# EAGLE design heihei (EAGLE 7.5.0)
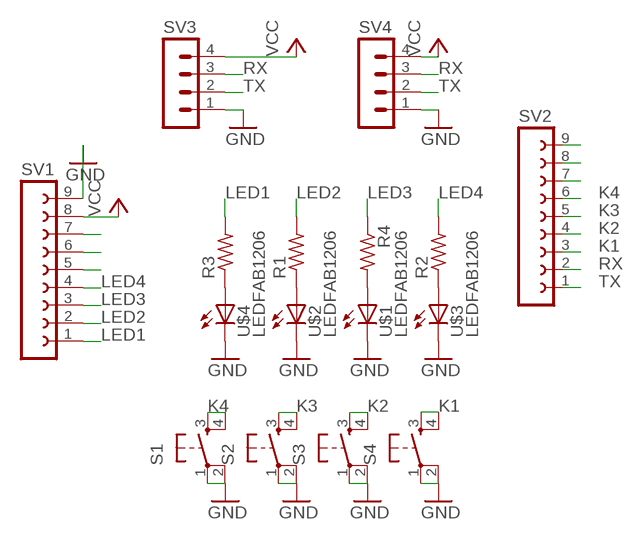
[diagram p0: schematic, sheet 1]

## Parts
R1  RES-US1206FAB  [R1206FAB]
R2  RES-US1206FAB  [R1206FAB]
R3  RES-US1206FAB  [R1206FAB]
R4  RES-US1206FAB  [R1206FAB]
S1  6MM_SWITCH6MM_SWITCH  [6MM_SWITCH]
S2  6MM_SWITCH6MM_SWITCH  [6MM_SWITCH]
S3  6MM_SWITCH6MM_SWITCH  [6MM_SWITCH]
S4  6MM_SWITCH6MM_SWITCH  [6MM_SWITCH]
SV1  FE09-1  [FE09]
SV2  FE09-1  [FE09]
SV3  MA04-1  [MA04-1]
SV4  MA04-1  [MA04-1]
U$1  LEDFAB1206  [LED1206FAB]
U$2  LEDFAB1206  [LED1206FAB]
U$3  LEDFAB1206  [LED1206FAB]
U$4  LEDFAB1206  [LED1206FAB]

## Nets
GND: S1.1(P) S1.2(P1) S2.1(P) S2.2(P1) S3.1(P) S3.2(P1) S4.1(P) S4.2(P1) SV1.9 SV3.1 SV4.1 U$1.2(C) U$2.2(C) U$3.2(C) U$4.2(C)
K1: S4.3(S) S4.4(S1) SV2.3
K2: S3.3(S) S3.4(S1) SV2.4
K3: S2.3(S) S2.4(S1) SV2.5
K4: S1.3(S) S1.4(S1) SV2.6
LED1: R3.2 SV1.1
LED2: R1.2 SV1.2
LED3: R4.1 SV1.3
LED4: R2.2 SV1.4
N$1: SV2.8
N$2: SV2.9
N$3: SV2.7
N$12: SV1.7
N$13: SV1.6
N$18: R3.1 U$4.1(A)
N$19: R1.1 U$2.1(A)
N$20: R4.2 U$1.1(A)
N$21: R2.1 U$3.1(A)
N$22: SV1.5
RX: SV2.2 SV3.3 SV4.3
TX: SV2.1 SV3.2 SV4.2
VCC: SV1.8 SV3.4 SV4.4

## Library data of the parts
R1-R4 = fab:RES-US: Resistor (US Symbol)
S1-S4 = fab:6MM_SWITCH: OMRON SWITCH
SV1 SV2 = con-lsta:FE09-1: FEMALE HEADER; OC_FARNELL: unknown; OC_NEWARK: unknown
SV3 SV4 = con-lstb:MA04-1: PIN HEADER; OC_FARNELL: unknown; OC_NEWARK: unknown
U$1-U$4 = fab:LED: LED

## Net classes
0 default: clearance 0.205 mm

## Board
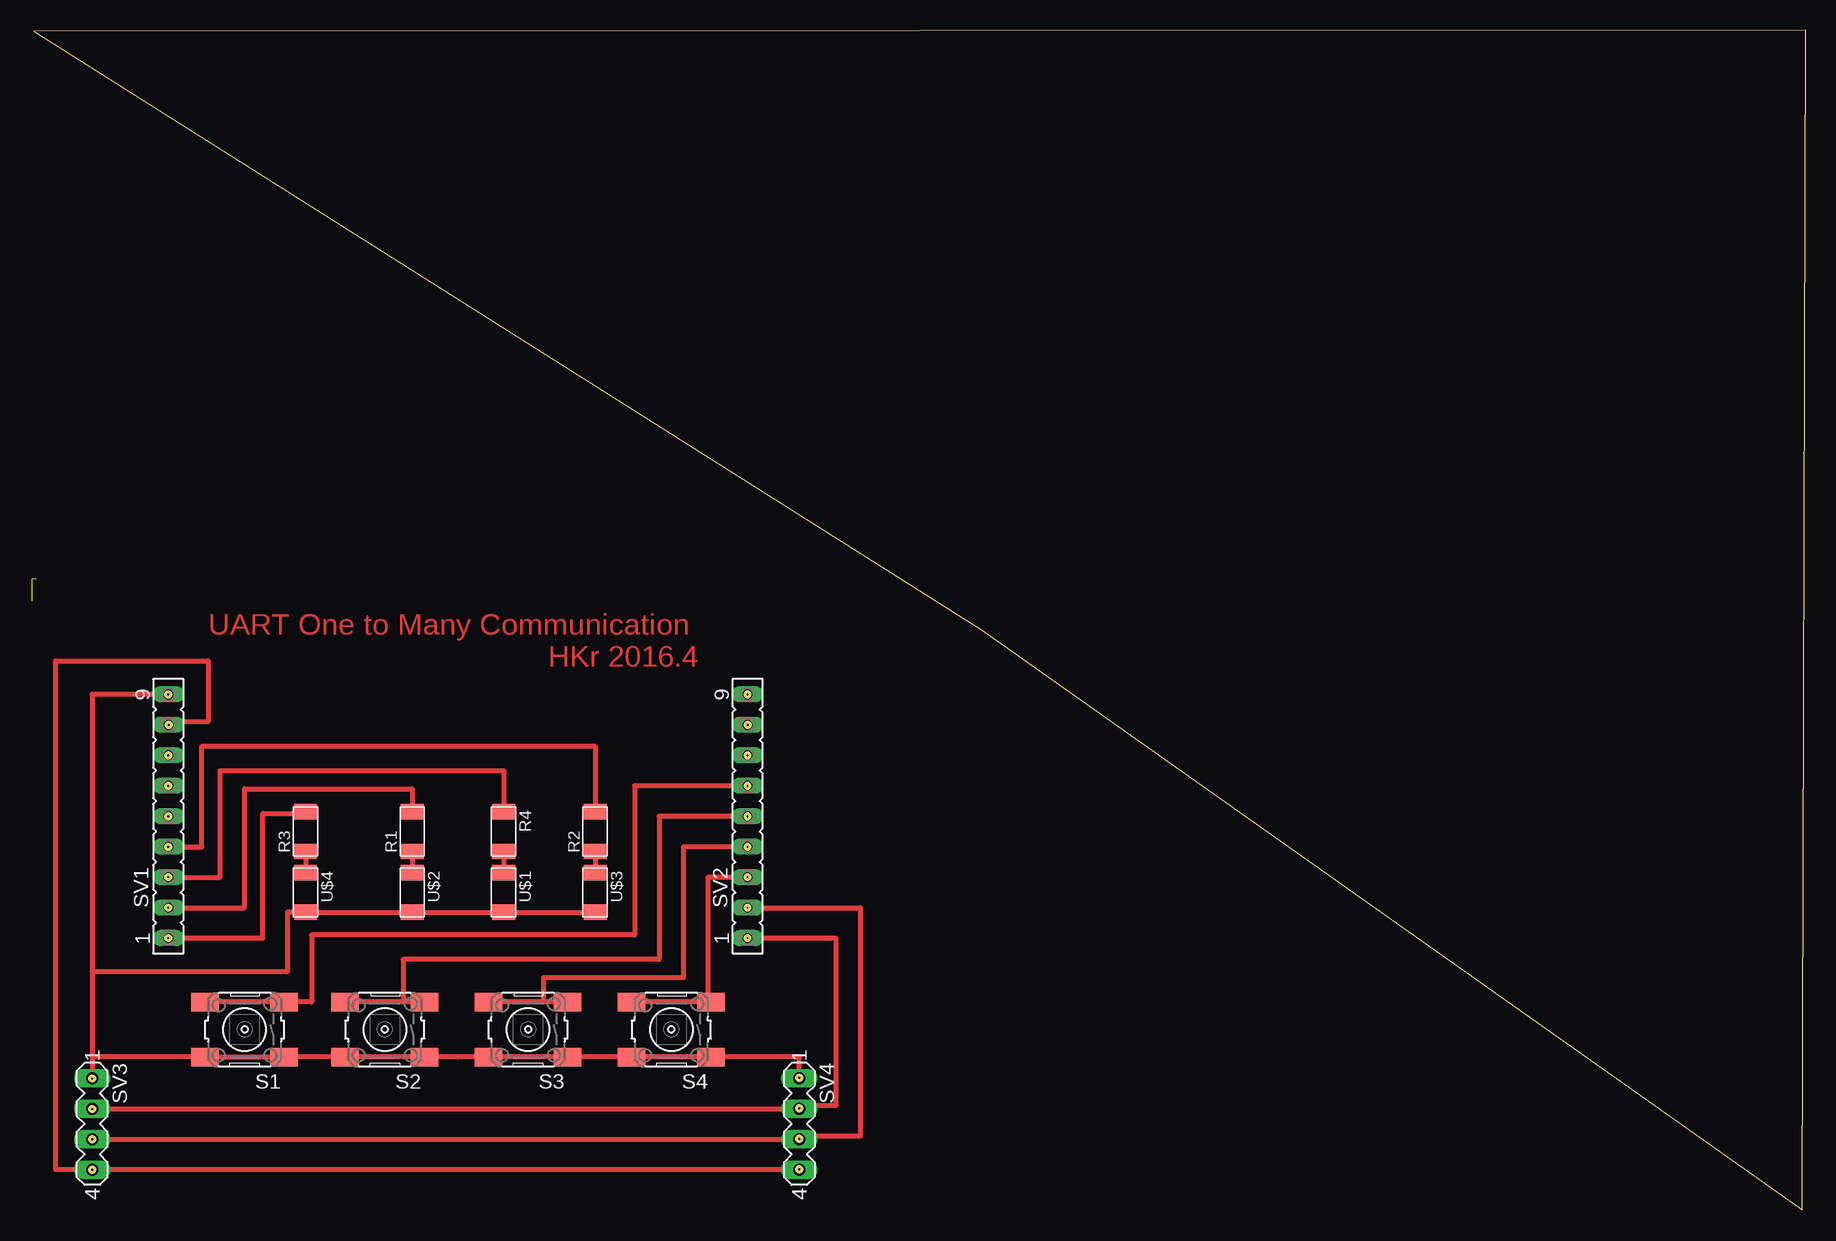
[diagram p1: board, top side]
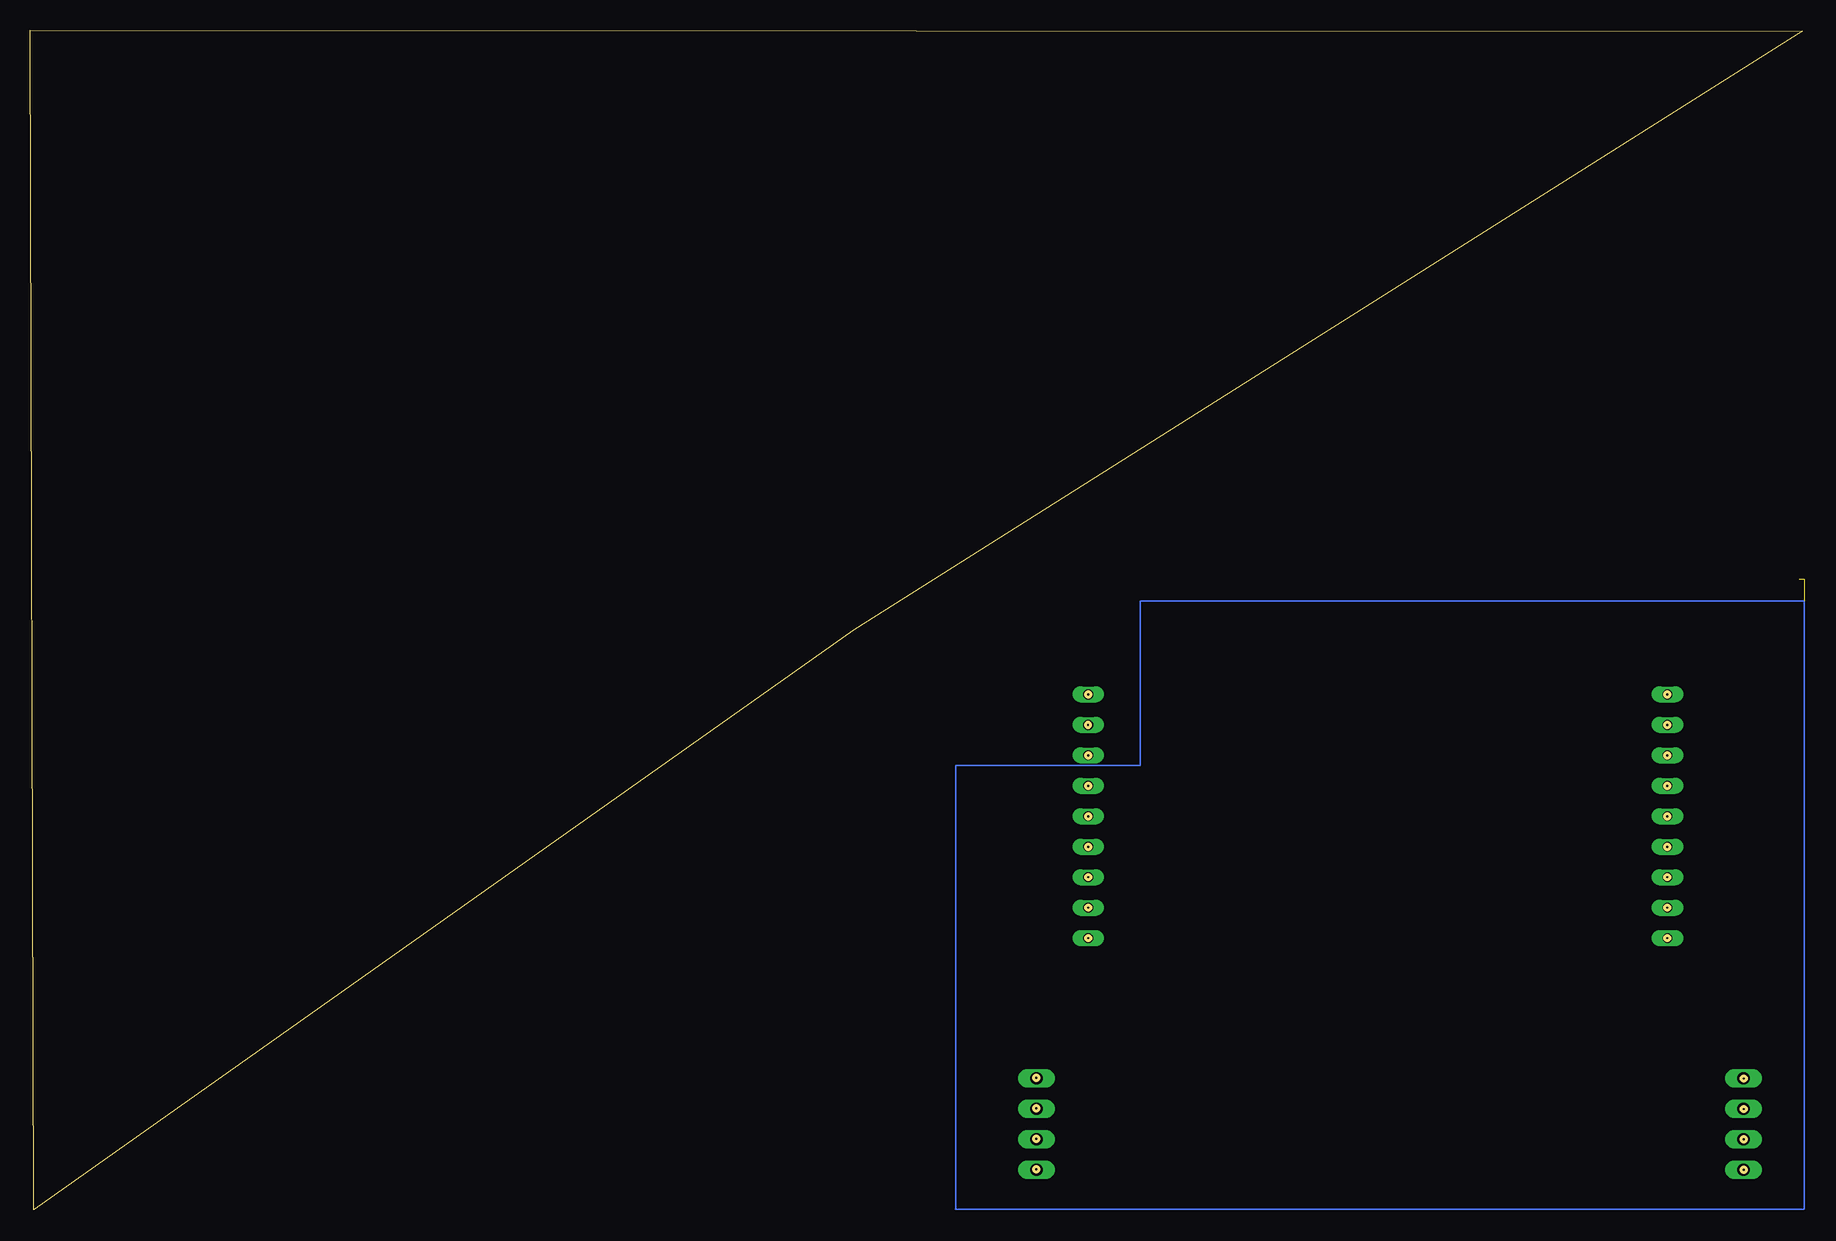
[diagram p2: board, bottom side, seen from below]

Size 147.68 x 98.36 mm. Coordinates in mm from the lower left corner, seen from the top.
Outline: 79.02,48.36 147.37,0 147.68,98.36 0,98.26 79.02,48.36
Copper layers (1*16): Top 0.035mm / dielectric 1.5mm / Bottom 0.035mm
Design rules "default": minimum track width 10mil, minimum drill 24mil, track to track 8mil, track to pad 8mil, pad to pad 8mil, via to via 8mil, smd to smd 8mil, copper to edge 40mil, drill to drill 8mil, minimum pad ring 10mil, minimum via ring 8mil, stop-mask expansion 4mil, vias tented up to drill 0mil, thermal gap 10mil
Milling: area 59.3,42.8 to 59.7,43.2; area 59.3,40.2 to 59.7,40.6; area 59.3,37.7 to 59.7,38.1; area 59.3,35.2 to 59.7,35.6; area 59.3,32.6 to 59.7,33; area 59.3,30.1 to 59.7,30.5; area 59.3,27.5 to 59.7,27.9; area 59.3,25 to 59.7,25.4; area 59.3,22.5 to 59.7,22.9; area 11,42.8 to 11.4,43.2; area 11,40.2 to 11.5,40.6; area 11,37.7 to 11.4,38.1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

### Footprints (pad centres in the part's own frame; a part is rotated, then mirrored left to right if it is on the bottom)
R1206FAB = smd 1.27 x 1.905: 1 -1.651,0; 2 1.651,0
6MM_SWITCH = smd 2.286 x 1.524: 1 -3.302,2.286; 2 3.302,2.286; 3 -3.302,-2.286; 4 3.302,-2.286
FE09 = drill 0.813 long: 1 -10.16,0; 2 -7.62,0; 3 -5.08,0; 4 -2.54,0; 5 0,0; 6 2.54,0; 7 5.08,0; 8 7.62,0; 9 10.16,0
MA04-1 = drill 1.016 long: 1 -3.81,0; 2 -1.27,0; 3 1.27,0; 4 3.81,0
LED1206FAB = smd 1.27 x 1.905: 1 -1.651,0; 2 1.651,0

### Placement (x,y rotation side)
R1  31.55,31.55 90 top
R2  46.79,31.55 90 top
R3  22.66,31.55 90 top
R4  39.17,31.55 270 top
S1  17.58,15.04 180 top
S2  29.26,15.04 180 top
S3  41.2,15.04 180 top
S4  53.14,15.04 180 top
SV1  11.23,32.82 90 top
SV2  59.49,32.82 90 top
SV3  4.88,7.16 270 top
SV4  63.8,7.16 270 top
U$1  39.17,26.47 270 top
U$2  31.55,26.47 270 top
U$3  46.79,26.47 270 top
U$4  22.66,26.47 270 top

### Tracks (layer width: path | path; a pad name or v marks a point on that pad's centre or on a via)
GND
  Top 0.406: U$3.2 U$1.2 U$2.2 U$4.2 21.13,24.82 21.13,19.86 4.88,19.86 | S4.1 S4.2 | S4.1 S3.1 S3.2 | S3.2 35.36,12.75 | S3.2 S2.1 S2.2 S1.1 S1.2 4.88,12.75 SV3.1 4.88,19.86 | SV1.9 4.88,42.98 4.88,19.86 | SV4.1 63.81,12.75 S4.1
K1
  Top 0.406: SV2.3 56.19,27.74 56.19,17.32 S4.3 S4.4
K2
  Top 0.406: SV2.4 54.15,30.28 54.15,19.35 42.47,19.35 42.47,17.32 | S3.3 42.47,17.32 | 42.47,17.32 S3.4
K3
  Top 0.406: SV2.5 52.12,32.82 52.12,20.88 30.79,20.88 30.79,17.32 | S2.3 30.79,17.32 | 30.79,17.32 S2.4
K4
  Top 0.406: S1.4 S1.3 23.17,17.32 23.17,22.91 50.09,22.91 50.09,35.36 SV2.6
LED1
  Top 0.406: SV1.1 19.1,22.66 19.1,33.07 22.66,33.07 R3.2
LED2
  Top 0.406: SV1.2 17.58,25.2 17.58,35.1 31.55,35.1 R1.2
LED3
  Top 0.406: SV1.3 15.55,27.74 15.55,36.63 39.17,36.63 R4.1
LED4
  Top 0.406: SV1.4 14.02,30.28 14.02,38.66 46.79,38.66 R2.2
N$6  (2 unrouted)
  Bottom 0.127: 70.54,0.05 -0.18,0.05 -0.18,50.75 55.17,50.75 55.17,37.03 70.54,37.03 70.54,0.05 | 70.59,0.05 70.54,0.05
N$18
  Top 0.406: R3.1 U$4.1
N$19
  Top 0.406: R1.1 U$2.1
N$20
  Top 0.406: R4.2 U$1.1
N$21
  Top 0.406: R2.1 U$3.1
RX
  Top 0.406: SV2.2 68.89,25.2 68.89,6.15 63.81,6.15 SV4.3 SV3.3
TX
  Top 0.406: SV2.1 66.85,22.66 66.85,8.69 63.81,8.69 SV4.2 SV3.2
VCC
  Top 0.406: SV1.8 11.23,40.69 14.53,40.69 14.53,45.77 1.83,45.77 1.83,3.35 SV3.4 SV4.4

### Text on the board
Top: UART One to Many Communication / HKr 2016.4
